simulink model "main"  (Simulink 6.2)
settings: Solver=ode4  StartTime=0.0  StopTime=20  FixedStep=.01  RelTol=1e-3

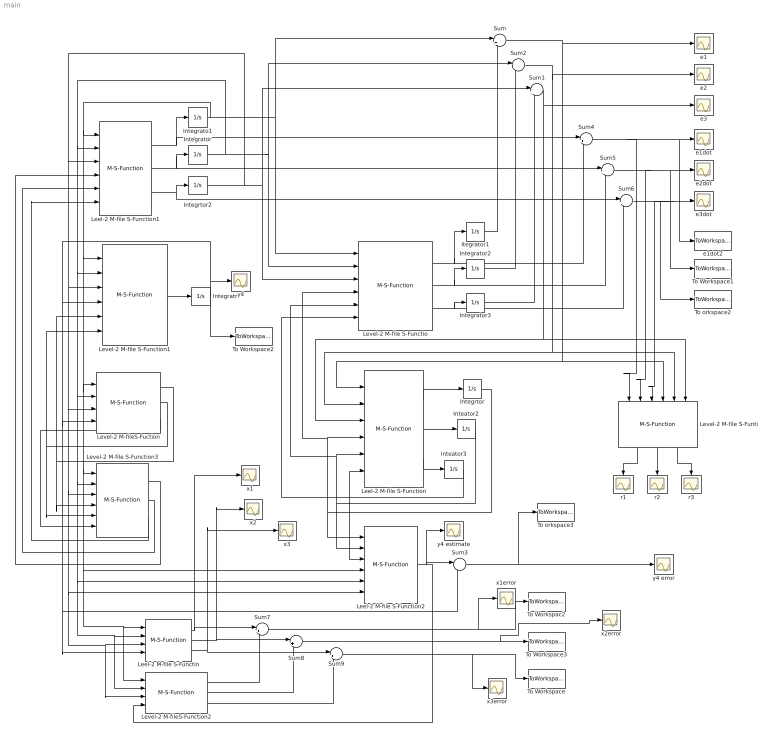
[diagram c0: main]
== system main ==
  Inteator2 : Integrator  InitialCondition=1
  Inteator3 : Integrator  InitialCondition=1
  Integrato1 : Integrator  InitialCondition=.769
  Integrator : Integrator  InitialCondition=1.15
  Integrator2 : Integrator  InitialCondition=1.15
  Integrator3 : Integrator  InitialCondition=1.92
  Integratr : Integrator  InitialCondition=1.92
  Integrtor : Integrator  InitialCondition=1
  Integrtor2 : Integrator  InitialCondition=1.92
  Itegrator1 : Integrator  InitialCondition=.769
  Leel-2 M-file S-Functin : M-S-Function  MFile=x_123
  Leel-2 M-file S-Function : M-S-Function  MFile=f_123estimate
  Leel-2 M-file S-Function1 : M-S-Function  MFile=y_dynamics123
  Leel-2 M-file S-Function2 : M-S-Function  MFile=y_4estimate
  Level-2 M-file S-Functio : M-S-Function  MFile=y_dynamics123estimate
  Level-2 M-file S-Function1 : M-S-Function  MFile=y_dynamics4
  Level-2 M-file S-Function3 : M-S-Function  MFile=f_123
  Level-2 M-file S-Funti : M-S-Function  Orientation=down  MFile=r_123
  Level-2 M-fileS-Fuction : M-S-Function  MFile=y_567
  Level-2 M-fileS-Function2 : M-S-Function  MFile=x_123estimate
  Sum{,1..2,4..9} (9 alike) : Sum  Inputs=|+-
  Sum3 : Sum  Inputs=|-+
  To Workspac2 : ToWorkspace  VariableName=x1error  SampleTime=-1  SaveFormat=Structure
  To Workspace : ToWorkspace  VariableName=x3error  SampleTime=-1  SaveFormat=Structure
  To Workspace1 : ToWorkspace  VariableName=e2dot  SampleTime=-1  SaveFormat=Array
  To Workspace2 : ToWorkspace  VariableName=y4  SampleTime=-1  SaveFormat=Array
  To Workspace3 : ToWorkspace  VariableName=x2error  SampleTime=-1  SaveFormat=Structure
  To orkspace2 : ToWorkspace  VariableName=e3dot  SampleTime=-1  SaveFormat=Array
  To orkspace3 : ToWorkspace  VariableName=y4error  SampleTime=-1  SaveFormat=Array
  e1 : Scope
  e1dot : Scope
  e1dot2 : ToWorkspace  VariableName=e1dot  SampleTime=-1  SaveFormat=Array
  e2 : Scope
  e2dot : Scope
  e3 : Scope
  e3dot : Scope
  r1 : Scope
  r2 : Scope
  r3 : Scope
  x1 : Scope
  x1error : Scope
  x2 : Scope
  x2error : Scope
  x3 : Scope
  x3error : Scope
  y4 : Scope
  y4 error : Scope
  y4 estimate : Scope
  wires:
  Leel-2 M-file S-Function1/1 -> Integrato1/1, Sum4/1
  Leel-2 M-file S-Function1/2 -> Sum5/1, Integrator/1
  Leel-2 M-file S-Function1/3 -> Integrtor2/1, Sum6/1
  Level-2 M-file S-Functio/1 -> Itegrator1/1, Sum4/2
  Level-2 M-file S-Functio/2 -> Integrator2/1, Sum5/2
  Level-2 M-file S-Functio/3 -> Integrator3/1, Sum6/2
  Itegrator1/1 -> Sum/2
  Integrator2/1 -> Sum2/2
  Integrator3/1 -> Sum1/2
  Sum1/1 -> e3/1, Leel-2 M-file S-Function/3, Level-2 M-file S-Funti/6
  Sum2/1 -> e2/1, Leel-2 M-file S-Function/2, Level-2 M-file S-Funti/5
  Sum/1 -> e1/1, Leel-2 M-file S-Function/1, Level-2 M-file S-Funti/4
  Leel-2 M-file S-Function/1 -> Integrtor/1
  Leel-2 M-file S-Function/2 -> Inteator2/1
  Leel-2 M-file S-Function/3 -> Inteator3/1
  Inteator3/1 -> Leel-2 M-file S-Function/6, Level-2 M-file S-Functio/6, Leel-2 M-file S-Function2/3
  Inteator2/1 -> Leel-2 M-file S-Function/5, Level-2 M-file S-Functio/5, Leel-2 M-file S-Function2/2
  Integrtor/1 -> Leel-2 M-file S-Function/4, Level-2 M-file S-Functio/4, Leel-2 M-file S-Function2/1
  Integrato1/1 -> Leel-2 M-file S-Function1/1, Level-2 M-file S-Function1/1, Level-2 M-fileS-Fuction/1, Level-2 M-file S-Function3/1, Leel-2 M-file S-Function2/4, Leel-2 M-file S-Functin/1, Level-2 M-fileS-Function2/1, Level-2 M-file S-Functio/1, Sum/1
  Integrator/1 -> Leel-2 M-file S-Function1/2, Level-2 M-file S-Function1/2, Level-2 M-fileS-Fuction/2, Level-2 M-file S-Function3/2, Leel-2 M-file S-Functin/2, Level-2 M-fileS-Function2/2, Leel-2 M-file S-Function2/5, Level-2 M-file S-Functio/2, Sum2/1
  Integrtor2/1 -> Leel-2 M-file S-Function1/3, Level-2 M-file S-Function1/3, Level-2 M-fileS-Fuction/3, Level-2 M-file S-Function3/3, Leel-2 M-file S-Function2/6, Leel-2 M-file S-Functin/3, Level-2 M-fileS-Function2/3, Level-2 M-file S-Functio/3, Sum1/1
  Sum4/1 -> Level-2 M-file S-Funti/1, e1dot/1, e1dot2/1
  Sum5/1 -> Level-2 M-file S-Funti/2, e2dot/1, To Workspace1/1
  Sum6/1 -> e3dot/1, Level-2 M-file S-Funti/3, To orkspace2/1
  Level-2 M-file S-Funti/1 -> r1/1
  Level-2 M-file S-Funti/2 -> r2/1
  Level-2 M-file S-Funti/3 -> r3/1
  Level-2 M-file S-Function1/1 -> Integratr/1
  Integratr/1 -> Level-2 M-file S-Function1/4, Level-2 M-fileS-Fuction/4, Sum3/2, Leel-2 M-file S-Functin/4, y4/1, To Workspace2/1
  Level-2 M-fileS-Fuction/3 -> Level-2 M-file S-Function3/6
  Level-2 M-fileS-Fuction/2 -> Level-2 M-file S-Function3/5, Level-2 M-file S-Function1/6
  Level-2 M-fileS-Fuction/1 -> Level-2 M-file S-Function3/4, Level-2 M-file S-Function1/5
  Level-2 M-file S-Function3/3 -> Leel-2 M-file S-Function1/6
  Level-2 M-file S-Function3/2 -> Leel-2 M-file S-Function1/5
  Level-2 M-file S-Function3/1 -> Leel-2 M-file S-Function1/4
  Leel-2 M-file S-Function2/1 -> Sum3/1, y4 estimate/1, Level-2 M-fileS-Function2/4
  Sum3/1 -> y4 error/1, To orkspace3/1
  Leel-2 M-file S-Functin/1 -> Sum7/1, x1/1
  Leel-2 M-file S-Functin/2 -> Sum8/1, x2/1
  Leel-2 M-file S-Functin/3 -> Sum9/1, x3/1
  Level-2 M-fileS-Function2/1 -> Sum7/2
  Level-2 M-fileS-Function2/2 -> Sum8/2
  Level-2 M-fileS-Function2/3 -> Sum9/2
  Sum7/1 -> To Workspac2/1, x1error/1
  Sum8/1 -> To Workspace3/1, x2error/1
  Sum9/1 -> To Workspace/1, x3error/1
